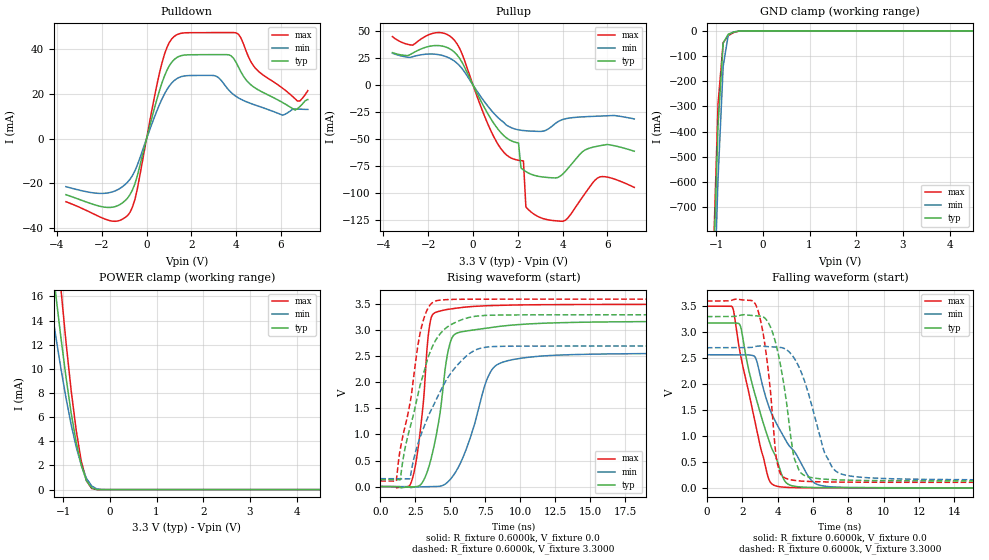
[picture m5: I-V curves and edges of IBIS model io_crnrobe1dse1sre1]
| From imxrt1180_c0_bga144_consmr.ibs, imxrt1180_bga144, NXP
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[Model]  io_crnrobe1dse1sre1
|   Model io_crnrobe1dse1sre1
| This model was characterised for following simulation conditions:
| External (pad) voltage:
|   - Typ: 3.3V,   - Min: 2.7V,   - Max: 3.6V
| Library cells for typ/min/max conditions are connected as defined below:
|  PAD_IO - External Pad
|  ipp_do - Core Input
|  ipp_obe - Output Buffer Enable
|  ASRCN3V3[3] - NC
|  ASRCN3V3[4] - NC
|  ASRCP3V3[4] - NC
|  REFAPBIAS3V3 - gnde
|  REFBAMPL3V3 - vdd1v8
|  REFCAMPH3V3 - vdd1v8
|  REFDNBIAS3V3 - vdd1v8
|  REFH3V3 - REFH3V3
|  REFL3V3 - REFL3V3
|  gnde - gnde
|  ipp_dse - vdd
|  ipp_ina235_3v - NC
|  ipp_ina40_3v - NC
|  ipp_ina_mux - NC
|  ipp_ind - NC
|  ipp_ind_1p8v - NC
|  ipp_ind_3v - NC
|  ipp_sre - vdd
|  vdd - vdd
|  vdd1v8 - vdd1v8
|  vdda - vdde3v3
|  vdde3v3 - vdde3v3
| All other pins connected to ground
Model_type I/O
Polarity   Non-Inverting
Enable   Active-High
Vinl =   0.9900V
Vinh =   2.3100V
Vmeas =  1.6500V
Cref =   15.0000pF
Rref =   0.6000k
Vref =   0.0V
C_comp   4.0038pF   3.8208pF   4.1229pF
|C_comp_pullup   0.5150pF   0.5958pF   0.4948pF
|C_comp_pulldown   2.0814pF   2.1736pF   1.8625pF
[Model Spec]
| variable   typ   min   max
Vinh   2.3100V   NA   NA
Vinl   0.9900V   NA   NA
Vref   0.0V   0.0V   0.0V
Cref   15.0000pF   15.0000pF   15.0000pF
Rref   0.6000k   0.6000k   0.6000k
[Receiver Thresholds]
Vcross_high  =   0.0V
Vcross_low  =   0.0V
Vdiff_ac  =   0.0V
Vdiff_dc  =   0.0V
Tdiffslew_ac  =   0.0S
[Temperature Range]   25.0000   0.1250k   -40.0000
[Voltage Range]   3.3000V   2.7000V   3.6000V
[Pullup Reference]   3.3000V   2.7000V   3.6000V
[Pulldown Reference]   0.0V   0.0V   0.0V
[POWER Clamp Reference]   3.3000V   2.7000V   3.6000V
[GND Clamp Reference]   0.0V   0.0V   0.0V
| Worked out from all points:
|   slope of the pulldown table from 0 to 0.495 V, typ, clamps not added: 26.5 ohm
|   slope of the pullup table from 0 to 0.495 V, typ, clamps not added: 24.3 ohm
|   GND clamp passes 1 mA (typ) near -0.49 V on its own axis
|   POWER clamp passes 1 mA (typ) near -0.52 V on its own axis
|   rising waveform, R_fixture 0.6000k, V_fixture 0.0: 20-80 % time 1.08ns typ, 1.78ns min, 706ps max; typ from 0 V to 3.18 V
|   rising waveform, R_fixture 0.6000k, V_fixture 3.3000: 20-80 % time 1.89ns typ, 2.56ns min, 1.33ns max; typ from 0.133 V to 3.3 V
|   falling waveform, R_fixture 0.6000k, V_fixture 0.0: 20-80 % time 1.65ns typ, 2.18ns min, 1.32ns max; typ from 3.18 V to 0 V
|   falling waveform, R_fixture 0.6000k, V_fixture 3.3000: 20-80 % time 855ps typ, 1.3ns min, 635ps max; typ from 3.3 V to 0.133 V
[Pulldown]
|Voltage   I(typ)   I(min)   I(max)
-3.6V     -24.99mA   -21.42mA   -28.15mA
-1.73V    -30.7mA    -24.22mA   -36.35mA
-740mV    -24.98mA   -18.14mA   -32.92mA
-410mV    -16.5mA    -11.77mA   -22.36mA
690mV     24.98mA    17.78mA    33.89mA
1.35V     36.27mA    26.82mA    46.47mA
3.11V     37.58mA    27.95mA    47.42mA
3.99V     34.3mA     18.95mA    47.34mA
5.09V     21.27mA    14.22mA    29.34mA
6.08V     16.14mA    10.5mA     22.54mA
6.74V     13.43mA    13.23mA    16.85mA
7.2V      17.5mA     13.09mA    21.48mA
[Pullup]
|Voltage   I(typ)   I(min)   I(max)
-3.6V     30.01mA    29.47mA    44.8mA
-2.7V     29.52mA    26.26mA    36.88mA
-830mV    30.4mA     22.17mA    41.43mA
1.04V     -38.71mA   -28.5mA    -52.1mA
2.03V     -53.47mA   -41.35mA   -69.49mA
2.14V     -76.57mA   -41.72mA   -69.82mA
2.25V     -78.4mA    -42mA      -70.06mA
2.36V     -79.96mA   -42.21mA   -112.7mA
2.69V     -83.13mA   -42.61mA   -118.9mA
4.12V     -79.83mA   -31.15mA   -125mA
5.66V     -56.09mA   -28.64mA   -84.82mA
7.2V      -61.13mA   -31.27mA   -94.53mA
[GND_clamp]
|Voltage   I(typ)   I(min)   I(max)
-3.6V     -19.67A    -19.55A    -20.65A
-1.07V    -1.013A    -1.224A    -956.3mA
-960mV    -377.1mA   -587.4mA   -291.7mA
-850mV    -48.2mA    -140.8mA   -46.94mA
-740mV    -13.57mA   -15.62mA   -19.22mA
-630mV    -5.136mA   -4.37mA    -7.235mA
-520mV    -1.276mA   -1.53mA    -1.554mA
-300mV    -4.356uA   -32.48uA   -995.7nA
7.2V      0A         0A         0A
[POWER_clamp]
|Voltage   I(typ)   I(min)   I(max)
-3.6V     102.7mA    81.65mA    131.1mA
-1.38V    23.95mA    18.52mA    31.78mA
-1.27V    20.01mA    15.56mA    26.56mA
-1.16V    16.22mA    12.73mA    21.52mA
-1.05V    12.64mA    10.07mA    16.71mA
-830mV    6.384mA    5.406mA    8.254mA
-720mV    3.9mA      3.518mA    4.888mA
-610mV    1.982mA    2.008mA    2.327mA
-500mV    727.2uA    927.8uA    733.5uA
-390mV    144.5uA    302.5uA    95.96uA
-170mV    198.4nA    4.047uA    20.3nA
7.2V      0A         0A         0A
[Ramp]
| variable   typ   min   max
dV/dt_r  1.9062/1.0759n   1.5391/1.7809n   2.1005/0.7056n
dV/dt_f  1.9001/0.8555n   1.5294/1.2969n   2.0958/0.6353n
R_load = 0.6000k
[Rising Waveform]
R_fixture= 0.6000k
V_fixture= 0.0
V_fixture_min= 0.0
V_fixture_max= 0.0
|time   V(typ)   V(min)   V(max)
0s        57.42nV    1.433uV    55.99nV
2.188ns   -7.802mV   -19.81mV   67.03mV
2.828ns   22.9mV     -5.641mV   1.009V
3.564ns   469.9mV    -2.893mV   3.167V
4.548ns   2.074V     32.98mV    3.39V
4.912ns   2.686V     112.6mV    3.407V
5.32ns    2.925V     254.3mV    3.422V
7.836ns   3.052V     2.186V     3.476V
9.789ns   3.11V      2.454V     3.488V
60ns      3.177V     2.565V     3.501V
[Rising Waveform]
R_fixture= 0.6000k
V_fixture= 3.3000
V_fixture_min= 2.7000
V_fixture_max= 3.6000
|time   V(typ)   V(min)   V(max)
0s        133.2mV    151mV      107mV
1.138ns   132.4mV    151mV      107.2mV
1.431ns   138.4mV    150.6mV    730.4mV
2.113ns   1.124V     153.3mV    1.591V
2.88ns    1.984V     979.2mV    2.995V
3.376ns   2.45V      1.321V     3.413V
4ns       2.832V     1.675V     3.57V
5.919ns   3.215V     2.451V     3.598V
8.033ns   3.292V     2.688V     3.599V
60ns      3.3V       2.7V       3.6V
[Falling Waveform]
R_fixture= 0.6000k
V_fixture= 0.0
V_fixture_min= 0.0
V_fixture_max= 0.0
|time   V(typ)   V(min)   V(max)
0s        3.177V     2.565V     3.501V
1.438ns   3.178V     2.565V     3.486V
1.871ns   3.14V      2.564V     2.624V
2.744ns   1.778V     2.511V     1.234V
3.442ns   989.4mV    1.633V     233.1mV
4.083ns   410.4mV    1.148V     23.3mV
4.596ns   71.19mV    841mV      8.132mV
5.913ns   7.853mV    145mV      1.293mV
7.089ns   2.924mV    18.31mV    366.4uV
60ns      1.076uV    4.112uV    889.6nV
[Falling Waveform]
R_fixture= 0.6000k
V_fixture= 3.3000
V_fixture_min= 2.7000
V_fixture_max= 3.6000
|time   V(typ)   V(min)   V(max)
0s        3.3V       2.7V       3.6V
2.753ns   3.316V     2.724V     3.536V
3.361ns   3.242V     2.723V     2.577V
3.968ns   2.691V     2.711V     497.8mV
4.859ns   724.9mV    2.54V      148.5mV
5.35ns    278.4mV    2.222V     130.3mV
6.703ns   166.4mV    644.6mV    114.3mV
7.299ns   155.6mV    322.2mV    111.7mV
8.305ns   145.9mV    218.4mV    109.4mV
60ns      133.2mV    151mV      107mV
